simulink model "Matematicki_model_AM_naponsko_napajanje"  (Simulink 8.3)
settings: Solver=ode3  StartTime=0  StopTime=Tfinalno  FixedStep=Tsim  RelTol=1e-3
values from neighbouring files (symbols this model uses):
  A1 = [-Rsigma/Lsigma 0 Lm/(Tr*Lr*Lsigma) 0; 0 -Rsigma/Lsigma 0 Lm/(Tr*Lr*Lsigma); Lm/Tr 0 -1/Tr 0; 0 Lm/Tr 0 -1/Tr]    [Matematicki_model_AM_naponsko_napajanje_parametri.m]
  A2 = [0 1 0 0; -1 0 0 0; 0 0 0 1; 0 0 -1 0]    [Matematicki_model_AM_naponsko_napajanje_parametri.m]
  A3 = [0 0 0 Lm/(Lr*Lsigma); 0 0 -Lm/(Lr*Lsigma) 0; 0 0 0 -1; 0 0 1 0]    [Matematicki_model_AM_naponsko_napajanje_parametri.m]
  Am = [-Kfv*p/J -Kel*p/J; 1 0]    [Matematicki_model_AM_naponsko_napajanje_parametri.m]
  B = [1/Lsigma 0; 0 1/Lsigma; 0 0; 0 0]    [Matematicki_model_AM_naponsko_napajanje_parametri.m]
  Bm = [p/J -p/J; 0 0]    [Matematicki_model_AM_naponsko_napajanje_parametri.m]
  Kp = 0.1    [Matematicki_model_AM_naponsko_napajanje_parametri.m]
  Lm = 0.422    [Matematicki_model_AM_naponsko_napajanje_parametri.m]
  Lr = Lxr+Lm    (= 0.462)    [Matematicki_model_AM_naponsko_napajanje_parametri.m]
  Lsigma = Ls*sigm    (= 0.0765367965368)    [Matematicki_model_AM_naponsko_napajanje_parametri.m]
  Mopt = 2    [Matematicki_model_AM_naponsko_napajanje_parametri.m]
  p = 2    [Matematicki_model_AM_naponsko_napajanje_parametri.m]
  Tn = 10*Tr    (= 0.733333333333)    [Matematicki_model_AM_naponsko_napajanje_parametri.m]
  topt = 1    [Matematicki_model_AM_naponsko_napajanje_parametri.m]
  TROUGAO_ZVEZDA = 0    [Matematicki_model_AM_naponsko_napajanje_parametri.m]
  Tsim = Tpwm/16    (= 3.125e-06)    [Matematicki_model_AM_naponsko_napajanje_parametri.m]
  U_f = Vm/ws    [Matematicki_model_AM_naponsko_napajanje_parametri.m]
  Vm = sqrt(2)*Veff    [Matematicki_model_AM_naponsko_napajanje_parametri.m]
  wk = 2*pi()*50    [Matematicki_model_AM_naponsko_napajanje_parametri.m]
  wref = ws    [Matematicki_model_AM_naponsko_napajanje_parametri.m]
  ws = 2*pi()*fs    [Matematicki_model_AM_naponsko_napajanje_parametri.m]
libraries: simulink x1

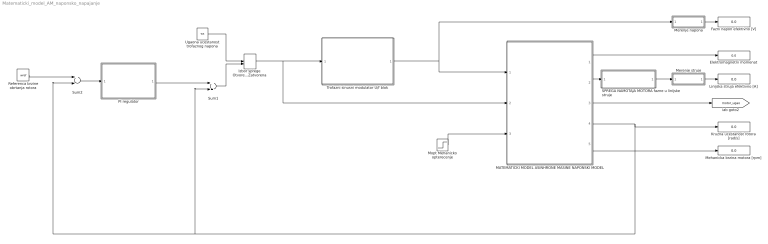
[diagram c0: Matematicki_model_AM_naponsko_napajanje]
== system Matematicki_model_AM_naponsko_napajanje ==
  Elektromagnetni momenat : Display
  Fazni napon efektivno [V] : Display
  Izbor sprege Otvorena / Zatvorena : ManualSwitch  CurrentSetting=0
  Kruzna ucestanost rotora [rad/s] : Display
  Linijska struja efektivno [A] : Display
  MATEMATICKI MODEL ASINHRONE MASINE NAPONSKI MODEL : Subsystem
  Mehanicka brzina motora [rpm] : Display
  Merenje napona : Subsystem
  Merenje struje : Subsystem
  Mopt Mehanicko opterecenje : Step  Time=4*topt  After=Mopt  SampleTime=Tsim
  PI regulator : Subsystem
  Referenca brzine obrtanja rotora : Constant  Value=wref  SampleTime=Tsim
  "SPREGA NAMOTAJA MOTORA fazne u linijske struje " : Subsystem
  Sum1 : Sum  SampleTime=Tsim
  Sum2 : Sum  Inputs=+-  SampleTime=Tsim
  Trofazni sinusni modulator U/f blok : Subsystem
  Ugaona ucestanost trofaznog napona : Constant  Value=ws  SampleTime=Tsim
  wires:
  Mopt Mehanicko opterecenje/1 -> MATEMATICKI MODEL ASINHRONE MASINE NAPONSKI MODEL/3(Mopt)
  MATEMATICKI MODEL ASINHRONE MASINE NAPONSKI MODEL/1(M_el) -> Elektromagnetni momenat/1
  MATEMATICKI MODEL ASINHRONE MASINE NAPONSKI MODEL/5(Brzina meh [o/min]) -> Mehanicka brzina motora [rpm]/1
  MATEMATICKI MODEL ASINHRONE MASINE NAPONSKI MODEL/3(ugao rot_el) -> [motor_ugao]
  Merenje napona/1(Us_eff) -> Fazni napon efektivno [V]/1
  Merenje struje/1(Is_eff) -> Linijska struja efektivno [A]/1
  "SPREGA NAMOTAJA MOTORA fazne u linijske struje "/1("Is_abc  invertor ") -> Merenje struje/1(Is_abc)
  MATEMATICKI MODEL ASINHRONE MASINE NAPONSKI MODEL/2(Is_abc) -> "SPREGA NAMOTAJA MOTORA fazne u linijske struje "/1(Is_abc fazno)
  MATEMATICKI MODEL ASINHRONE MASINE NAPONSKI MODEL/4(wr_el) -> Sum1/2, Sum2/2, Kruzna ucestanost rotora [rad/s]/1
  Ugaona ucestanost trofaznog napona/1 -> Izbor sprege Otvorena / Zatvorena/1
  Izbor sprege Otvorena / Zatvorena/1 -> MATEMATICKI MODEL ASINHRONE MASINE NAPONSKI MODEL/2(W_dq), Trofazni sinusni modulator U/f blok/1(ws)
  Sum1/1 -> Izbor sprege Otvorena / Zatvorena/2
  Referenca brzine obrtanja rotora/1 -> Sum2/1
  Sum2/1 -> PI regulator/1(e)
  PI regulator/1(wk) -> Sum1/1
  Trofazni sinusni modulator U/f blok/1(PWM) -> Merenje napona/1(Us_abc), MATEMATICKI MODEL ASINHRONE MASINE NAPONSKI MODEL/1(Us_abc)

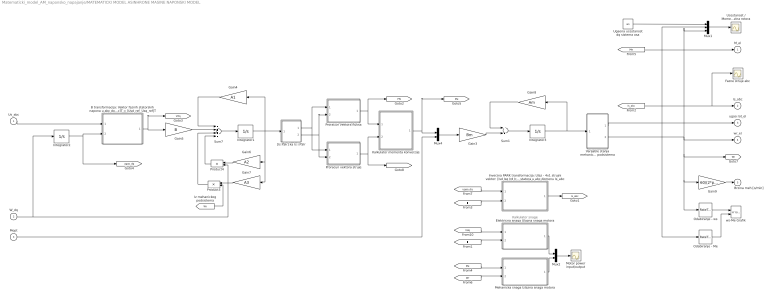
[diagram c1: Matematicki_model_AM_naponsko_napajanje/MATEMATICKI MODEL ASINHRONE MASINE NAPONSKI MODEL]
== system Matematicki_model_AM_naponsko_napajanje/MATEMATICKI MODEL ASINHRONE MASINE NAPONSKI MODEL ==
  note: Kalkulator snage
  Us_abc : Inport
  W_dq : Inport  Port=2
  Mopt : Inport  Port=3
  B transformacija: Vektor faznih statorskih napona u abc domenu u vektor napona u dq referentnom sistemu - [Usa  Usb Usc]T = [Usd_ref  Usq_ref]T : Subsystem
  Elektricna snaga Ulazna snaga motora : Subsystem
  Fazne struje abc : Scope
  Gain3 : Gain  Gain=Bm  Multiplication=Matrix(K*u) (u vector)  SampleTime=Tsim
  Gain4 : Gain  Gain=A1  Multiplication=Matrix(K*u) (u vector)  SampleTime=Tsim
  Gain5 : Gain  Gain=B  Multiplication=Matrix(K*u) (u vector)  SampleTime=Tsim
  Gain6 : Gain  Gain=A2  Multiplication=Matrix(K*u) (u vector)  SampleTime=Tsim
  Gain7 : Gain  Gain=A3  Multiplication=Matrix(K*u) (u vector)  SampleTime=Tsim
  Gain8 : Gain  Gain=Am  Multiplication=Matrix(K*u) (u vector)  SampleTime=Tsim
  Gain9 : Gain  Gain=60/(2*pi()*p)  SampleTime=Tsim
  Integrator1 : Integrator  InitialCondition=[0,0,0,0]
  Integrator2 : Integrator
  Integrator3 : Integrator  InitialCondition=[0,0]
  Inverzna PARK transformacija: Ulaz - 4x1 strujni vektor: [Isd Isq Ird Irq]T Izlaz - vektor struje statora u abc domenu Is_abc : Subsystem
  Kalkulator momenta konverzije : Subsystem
  Mehanicka snaga Izlazna snaga motora : Subsystem
  Motor power input/output : Scope
  Mux1 : Mux  Inputs=3
  Mux2 : Mux  Inputs=2
  Mux4 : Mux  Inputs=2
  Odabiranje - Me : RateTransition  OutPortSampleTime=100*Tsim
  Odabiranje - ws : RateTransition  OutPortSampleTime=100*Tsim
  Product3 : Product  SampleTime=Tsim
  Product4 : Product  SampleTime=Tsim
  Proracun vektora fluksa : Subsystem
  Proracun vektora struje : Subsystem
  Sum1 : Sum  SampleTime=Tsim
  Sum7 : Sum  Inputs=++++  SampleTime=Tsim
  Ucestanost / Momenat / Brzina rotora : Scope
  Ugaona ucestanost dq sistema osa : Constant  Value=ws  SampleTime=Tsim
  Varijable stanja mehanickog podsistema : Subsystem
  "[Is PSIr] ka Is i PSIr" : Subsystem
  ws-Me Grafik : simulink/Sinks/XY Graph  xmin=-400  xmax=400  ymin=-20  ymax=20  st=100*Tsim
  M_el : Outport  InitialOutput=0
  Is_abc : Outport  Port=2  InitialOutput=0
  ugao rot_el : Outport  Port=3  InitialOutput=0
  wr_el : Outport  Port=4  InitialOutput=0
  Brzina meh [o/min] : Outport  Port=5  InitialOutput=0
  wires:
  Us_abc/1 -> B transformacija: Vektor faznih statorskih napona u abc domenu u vektor napona u dq referentnom sistemu - [Usa  Usb Usc]T = [Usd_ref  Usq_ref]T/1(Us_abc)
  Integrator1/1 -> Gain4/1, Gain7/1, Gain6/1, "[Is PSIr] ka Is i PSIr"/1(X1)
  [Wr] -> Product3/2
  Product3/1 -> Sum7/3
  Gain7/1 -> Product3/1
  Gain6/1 -> Product4/1
  Sum7/1 -> Integrator1/1
  Gain4/1 -> Sum7/1
  Gain5/1 -> Sum7/2
  W_dq/1 -> Integrator2/1, Product4/2
  Integrator2/1 -> [ugao_dq], B transformacija: Vektor faznih statorskih napona u abc domenu u vektor napona u dq referentnom sistemu - [Usa  Usb Usc]T = [Usd_ref  Usq_ref]T/2(ugao_dq)
  [I] -> Inverzna PARK transformacija: Ulaz - 4x1 strujni vektor: [Isd Isq Ird Irq]T Izlaz - vektor struje statora u abc domenu Is_abc/2(I)
  B transformacija: Vektor faznih statorskih napona u abc domenu u vektor napona u dq referentnom sistemu - [Usa  Usb Usc]T = [Usd_ref  Usq_ref]T/1(Us_dq) -> Gain5/1, [Vdq]
  [I] -> Elektricna snaga Ulazna snaga motora/2(Is_dq)
  Elektricna snaga Ulazna snaga motora/1(Pel) -> Mux2/1
  [Me] -> Mehanicka snaga Izlazna snaga motora/1(Me)
  [Wr] -> Mehanicka snaga Izlazna snaga motora/2(Wr)
  Mux2/1 -> Motor power input/output/1
  Mehanicka snaga Izlazna snaga motora/1(Pmeh) -> Mux2/2
  [Vdq] -> Elektricna snaga Ulazna snaga motora/1(Vs_dq)
  Product4/1 -> Sum7/4
  "[Is PSIr] ka Is i PSIr"/1(Is) -> Proracun vektora struje/1(Is), Proracun vektora fluksa/1(Is)
  "[Is PSIr] ka Is i PSIr"/2(PSIr) -> Proracun vektora struje/2(PSIr), Proracun vektora fluksa/2(PSIr)
  Proracun vektora fluksa/1(PSI) -> [PSI], Kalkulator momenta konverzije/1(PSI)
  Proracun vektora struje/1(I) -> [I], Kalkulator momenta konverzije/2(I)
  Kalkulator momenta konverzije/1(Me) -> [Me], Mux4/1
  Mopt/1 -> Mux4/2
  [Me] -> M_el/1, Mux1/2, Odabiranje - Me/1
  Varijable stanja mehanickog podsistema/1(theta) -> ugao rot_el/1
  Varijable stanja mehanickog podsistema/2(w) -> Odabiranje - ws/1, Gain9/1, [Wr], wr_el/1, Mux1/3
  Gain9/1 -> Brzina meh [o/min]/1
  Inverzna PARK transformacija: Ulaz - 4x1 strujni vektor: [Isd Isq Ird Irq]T Izlaz - vektor struje statora u abc domenu Is_abc/1(Is_abc) -> [Is_abc]
  Mux4/1 -> Gain3/1
  Gain3/1 -> Sum1/2
  Sum1/1 -> Integrator3/1
  Gain8/1 -> Sum1/1
  Integrator3/1 -> Varijable stanja mehanickog podsistema/1(X2), Gain8/1
  [Is_abc] -> Is_abc/1, Fazne struje abc/1
  [ugao_dq] -> Inverzna PARK transformacija: Ulaz - 4x1 strujni vektor: [Isd Isq Ird Irq]T Izlaz - vektor struje statora u abc domenu Is_abc/1(ugao_dq)
  Mux1/1 -> Ucestanost / Momenat / Brzina rotora/1
  Odabiranje - ws/1 -> ws-Me Grafik/1
  Odabiranje - Me/1 -> ws-Me Grafik/2
  Ugaona ucestanost dq sistema osa/1 -> Mux1/1

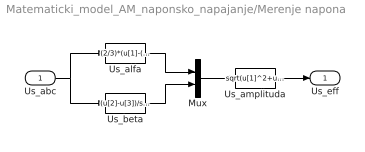
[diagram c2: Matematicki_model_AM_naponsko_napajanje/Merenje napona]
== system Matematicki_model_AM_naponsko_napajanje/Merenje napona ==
  Us_abc : Inport
  Mux : Mux  Inputs=2
  Us_alfa : Fcn  Expr=(2/3)*(u[1]-(u[2]+u[3])/2)  SampleTime=Tsim
  Us_amplituda : Fcn  Expr=sqrt(u[1]^2+u[2]^2)  SampleTime=Tsim
  Us_beta : Fcn  Expr=(u[2]-u[3])/sqrt(3)  SampleTime=Tsim
  Us_eff : Outport
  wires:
  Us_abc/1 -> Us_beta/1, Us_alfa/1
  Us_alfa/1 -> Mux/1
  Us_beta/1 -> Mux/2
  Mux/1 -> Us_amplituda/1
  Us_amplituda/1 -> Us_eff/1

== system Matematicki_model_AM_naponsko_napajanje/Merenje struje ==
  Is_abc : Inport
  Is_alfa : Fcn  Expr=(2/3)*(u[1]-(u[2]+u[3])/2)  SampleTime=Tsim
  Is_amplituda : Fcn  Expr=sqrt(u[1]^2+u[2]^2)/sqrt(2)  SampleTime=Tsim
  Is_beta : Fcn  Expr=(u[2]-u[3])/sqrt(3)  SampleTime=Tsim
  Mux : Mux  Inputs=2
  Is_eff : Outport
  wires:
  Is_amplituda/1 -> Is_eff/1
  Mux/1 -> Is_amplituda/1
  Is_beta/1 -> Mux/2
  Is_alfa/1 -> Mux/1
  Is_abc/1 -> Is_alfa/1, Is_beta/1

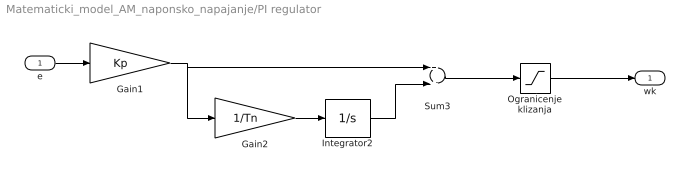
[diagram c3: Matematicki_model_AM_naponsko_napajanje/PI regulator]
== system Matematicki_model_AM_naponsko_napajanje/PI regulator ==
  e : Inport
  Gain1 : Gain  Gain=Kp  SampleTime=Tsim
  Gain2 : Gain  Gain=1/Tn  SampleTime=Tsim
  Integrator2 : Integrator  InitialCondition=[0]
  Ogranicenje klizanja : Saturate  UpperLimit=wk  LowerLimit=-wk  SampleTime=Tsim
  Sum3 : Sum  SampleTime=Tsim
  wk : Outport
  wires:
  Gain1/1 -> Sum3/1, Gain2/1
  e/1 -> Gain1/1
  Sum3/1 -> Ogranicenje klizanja/1
  Integrator2/1 -> Sum3/2
  Gain2/1 -> Integrator2/1
  Ogranicenje klizanja/1 -> wk/1

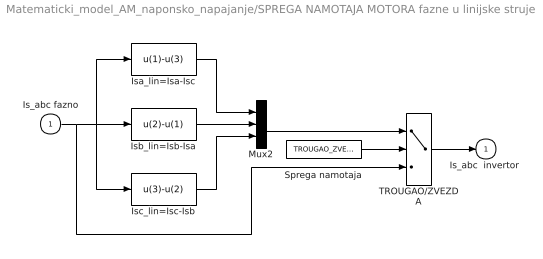
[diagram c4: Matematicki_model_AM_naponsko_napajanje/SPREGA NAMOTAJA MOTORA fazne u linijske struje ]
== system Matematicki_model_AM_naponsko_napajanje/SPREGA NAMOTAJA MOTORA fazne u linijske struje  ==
  Is_abc fazno : Inport
  Isa_lin=Isa-Isc : Fcn  Expr=u(1)-u(3)  SampleTime=Tsim
  Isb_lin=Isb-Isa : Fcn  Expr=u(2)-u(1)  SampleTime=Tsim
  Isc_lin=Isc-Isb : Fcn  Expr=u(3)-u(2)  SampleTime=Tsim
  Mux2 : Mux  Inputs=3
  Sprega namotaja : Constant  Value=TROUGAO_ZVEZDA
  TROUGAO/ZVEZDA : Switch  Threshold=0.1  SampleTime=Tsim
  "Is_abc  invertor " : Outport  InitialOutput=0
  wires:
  Isc_lin=Isc-Isb/1 -> Mux2/3
  Isb_lin=Isb-Isa/1 -> Mux2/2
  Isa_lin=Isa-Isc/1 -> Mux2/1
  Is_abc fazno/1 -> Isc_lin=Isc-Isb/1, Isb_lin=Isb-Isa/1, Isa_lin=Isa-Isc/1, TROUGAO/ZVEZDA/3
  TROUGAO/ZVEZDA/1 -> "Is_abc  invertor "/1
  Mux2/1 -> TROUGAO/ZVEZDA/1
  Sprega namotaja/1 -> TROUGAO/ZVEZDA/2

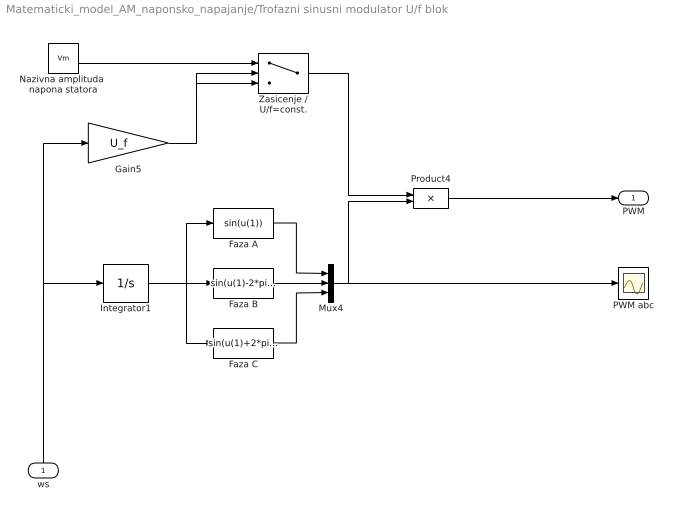
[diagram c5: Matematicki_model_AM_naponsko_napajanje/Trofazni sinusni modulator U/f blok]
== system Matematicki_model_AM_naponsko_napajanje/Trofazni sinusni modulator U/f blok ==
  ws : Inport
  Faza A : Fcn  Expr=sin(u(1))  SampleTime=Tsim
  Faza B : Fcn  Expr=sin(u(1)-2*pi()/3)  SampleTime=Tsim
  Faza C : Fcn  Expr=sin(u(1)+2*pi()/3)  SampleTime=Tsim
  Gain5 : Gain  Gain=U_f  SampleTime=Tsim
  Integrator1 : Integrator  InitialCondition=[0]
  Mux4 : Mux  Inputs=3
  Nazivna amplituda  napona statora : Constant  Value=Vm  SampleTime=Tsim
  PWM abc : Scope
  Product4 : Product  SampleTime=Tsim
  Zasicenje / U/f=const. : Switch  Criteria=u2 > Threshold  Threshold=Vm  SampleTime=Tsim
  PWM : Outport
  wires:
  Faza B/1 -> Mux4/2
  Faza A/1 -> Mux4/1
  Faza C/1 -> Mux4/3
  Gain5/1 -> Zasicenje / U/f=const./3, Zasicenje / U/f=const./2
  Nazivna amplituda  napona statora/1 -> Zasicenje / U/f=const./1
  Mux4/1 -> Product4/2, PWM abc/1
  Zasicenje / U/f=const./1 -> Product4/1
  Product4/1 -> PWM/1
  ws/1 -> Integrator1/1, Gain5/1
  Integrator1/1 -> Faza C/1, Faza B/1, Faza A/1

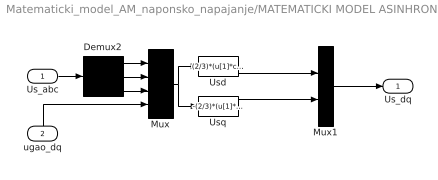
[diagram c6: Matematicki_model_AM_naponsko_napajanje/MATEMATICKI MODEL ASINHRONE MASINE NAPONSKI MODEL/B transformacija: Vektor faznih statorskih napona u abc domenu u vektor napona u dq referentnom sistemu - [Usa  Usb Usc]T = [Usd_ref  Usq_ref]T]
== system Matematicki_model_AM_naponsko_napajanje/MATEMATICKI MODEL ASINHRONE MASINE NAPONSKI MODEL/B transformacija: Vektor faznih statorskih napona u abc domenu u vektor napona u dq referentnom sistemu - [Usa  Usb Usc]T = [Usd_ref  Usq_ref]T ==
  Us_abc : Inport
  ugao_dq : Inport  Port=2
  Demux2 : Demux  Outputs=3
  Mux : Mux
  Mux1 : Mux  Inputs=2
  Usd : Fcn  Expr=(2/3)*(u[1]*cos(u[4])+u[2]*cos(u[4]-2*pi/3)+u[3]*cos(u[4]-4*pi/3))  SampleTime=Tsim
  Usq : Fcn  Expr=-(2/3)*(u[1]*sin(u[4])+u[2]*sin(u[4]-2*pi/3)+u[3]*sin(u[4]-4*pi/3))  SampleTime=Tsim
  Us_dq : Outport
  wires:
  Usd/1 -> Mux1/1
  Usq/1 -> Mux1/2
  Mux/1 -> Usq/1, Usd/1
  Demux2/2 -> Mux/2
  Demux2/3 -> Mux/3
  Demux2/1 -> Mux/1
  ugao_dq/1 -> Mux/4
  Us_abc/1 -> Demux2/1
  Mux1/1 -> Us_dq/1

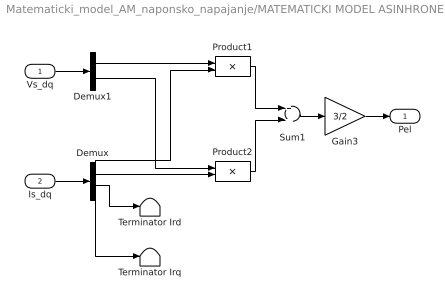
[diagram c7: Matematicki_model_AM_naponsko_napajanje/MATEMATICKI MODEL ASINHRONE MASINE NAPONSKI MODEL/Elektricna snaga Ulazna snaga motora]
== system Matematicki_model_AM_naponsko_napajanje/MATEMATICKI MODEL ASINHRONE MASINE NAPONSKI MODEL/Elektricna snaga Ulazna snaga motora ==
  Vs_dq : Inport
  Is_dq : Inport  Port=2
  Demux : Demux
  Demux1 : Demux  Outputs=2
  Gain3 : Gain  Gain=3/2  SampleTime=Tsim
  Product1 : Product  SampleTime=Tsim
  Product2 : Product  SampleTime=Tsim
  Sum1 : Sum  SampleTime=Tsim
  Terminator Ird : Terminator
  Terminator Irq : Terminator
  Pel : Outport
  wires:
  Sum1/1 -> Gain3/1
  Product2/1 -> Sum1/2
  Product1/1 -> Sum1/1
  Demux/2 -> Product2/2
  Demux1/2 -> Product2/1
  Demux/1 -> Product1/2
  Demux1/1 -> Product1/1
  Demux/3 -> Terminator Ird/1
  Demux/4 -> Terminator Irq/1
  Vs_dq/1 -> Demux1/1
  Gain3/1 -> Pel/1
  Is_dq/1 -> Demux/1

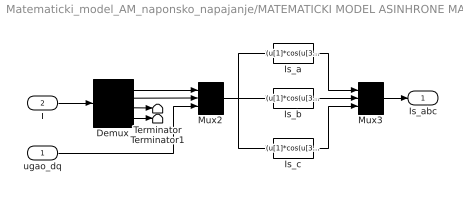
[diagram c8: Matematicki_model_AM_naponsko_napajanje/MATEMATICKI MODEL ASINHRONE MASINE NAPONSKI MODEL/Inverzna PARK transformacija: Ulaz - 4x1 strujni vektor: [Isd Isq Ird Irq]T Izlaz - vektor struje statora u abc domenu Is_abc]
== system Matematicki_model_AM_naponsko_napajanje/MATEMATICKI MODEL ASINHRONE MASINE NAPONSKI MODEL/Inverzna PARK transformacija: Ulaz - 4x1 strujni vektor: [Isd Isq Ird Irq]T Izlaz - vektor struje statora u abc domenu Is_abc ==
  ugao_dq : Inport
  I : Inport  Port=2
  Demux : Demux
  Is_a : Fcn  Expr=(u[1]*cos(u[3])-u[2]*sin(u[3]))  SampleTime=Tsim
  Is_b : Fcn  Expr=(u[1]*cos(u[3]-2*pi/3)-u[2]*sin(u[3]-2*pi/3))  SampleTime=Tsim
  Is_c : Fcn  Expr=(u[1]*cos(u[3]-4*pi/3)-u[2]*sin(u[3]-4*pi/3))  SampleTime=Tsim
  Mux2 : Mux  Inputs=3
  Mux3 : Mux  Inputs=3
  Terminator : Terminator
  Terminator1 : Terminator
  Is_abc : Outport
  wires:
  ugao_dq/1 -> Mux2/3
  Mux3/1 -> Is_abc/1
  I/1 -> Demux/1
  Mux2/1 -> Is_c/1, Is_a/1, Is_b/1
  Is_a/1 -> Mux3/1
  Is_b/1 -> Mux3/2
  Is_c/1 -> Mux3/3
  Demux/3 -> Terminator/1
  Demux/4 -> Terminator1/1
  Demux/1 -> Mux2/1
  Demux/2 -> Mux2/2

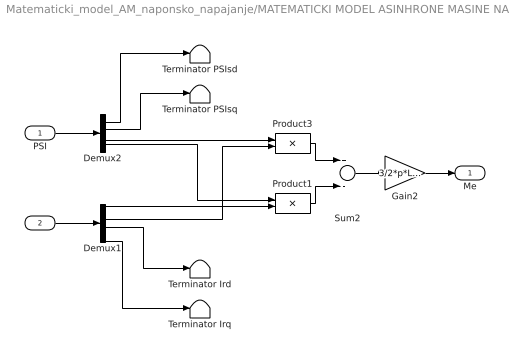
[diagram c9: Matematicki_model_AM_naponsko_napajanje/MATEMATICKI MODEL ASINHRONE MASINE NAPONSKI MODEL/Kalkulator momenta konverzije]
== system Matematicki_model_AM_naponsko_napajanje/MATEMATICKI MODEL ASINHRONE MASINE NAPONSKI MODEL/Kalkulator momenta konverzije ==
  PSI : Inport
  I : Inport  Port=2
  Demux1 : Demux
  Demux2 : Demux
  Gain2 : Gain  Gain=3/2*p*Lm/Lr  SampleTime=Tsim
  Product1 : Product  SampleTime=Tsim
  Product3 : Product  SampleTime=Tsim
  Sum2 : Sum  Inputs=+-  SampleTime=Tsim
  Terminator Ird : Terminator
  Terminator Irq : Terminator
  Terminator PSIsd : Terminator
  Terminator PSIsq : Terminator
  Me : Outport
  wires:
  PSI/1 -> Demux2/1
  Demux2/1 -> Terminator PSIsd/1
  Demux2/2 -> Terminator PSIsq/1
  Demux1/1 -> Product1/2
  Demux1/2 -> Product3/2
  I/1 -> Demux1/1
  Demux2/4 -> Product1/1
  Demux2/3 -> Product3/1
  Product3/1 -> Sum2/1
  Product1/1 -> Sum2/2
  Gain2/1 -> Me/1
  Sum2/1 -> Gain2/1
  Demux1/3 -> Terminator Ird/1
  Demux1/4 -> Terminator Irq/1

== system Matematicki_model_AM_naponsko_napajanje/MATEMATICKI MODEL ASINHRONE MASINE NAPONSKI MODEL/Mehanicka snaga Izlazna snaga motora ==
  note: Pmeh=Mel*Wr_el/P
  Me : Inport
  Wr : Inport  Port=2
  Gain11 : Gain  Gain=1/p  SampleTime=Tsim
  Product6 : Product  SampleTime=Tsim
  Pmeh : Outport
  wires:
  Product6/1 -> Gain11/1
  Me/1 -> Product6/1
  Gain11/1 -> Pmeh/1
  Wr/1 -> Product6/2

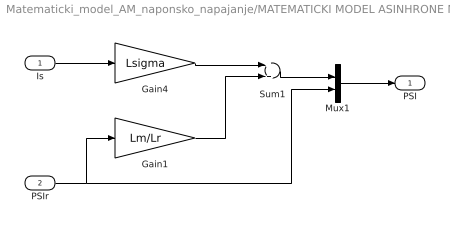
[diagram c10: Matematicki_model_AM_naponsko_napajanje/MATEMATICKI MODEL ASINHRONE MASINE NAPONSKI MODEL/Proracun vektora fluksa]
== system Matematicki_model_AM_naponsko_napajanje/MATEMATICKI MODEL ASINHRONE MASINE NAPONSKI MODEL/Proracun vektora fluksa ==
  Is : Inport
  PSIr : Inport  Port=2
  Gain1 : Gain  Gain=Lm/Lr  SampleTime=Tsim
  Gain4 : Gain  Gain=Lsigma  SampleTime=Tsim
  Mux1 : Mux  Inputs=2
  Sum1 : Sum  SampleTime=Tsim
  PSI : Outport
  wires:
  Is/1 -> Gain4/1
  Mux1/1 -> PSI/1
  PSIr/1 -> Gain1/1, Mux1/2
  Gain1/1 -> Sum1/2
  Gain4/1 -> Sum1/1
  Sum1/1 -> Mux1/1

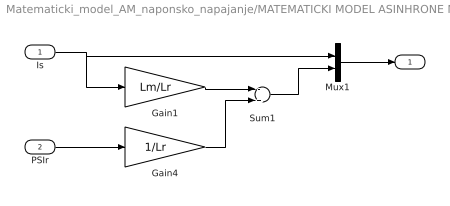
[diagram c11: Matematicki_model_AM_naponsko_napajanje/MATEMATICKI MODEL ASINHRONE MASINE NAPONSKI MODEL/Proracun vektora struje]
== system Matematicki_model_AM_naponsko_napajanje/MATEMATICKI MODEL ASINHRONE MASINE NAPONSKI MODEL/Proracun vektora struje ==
  Is : Inport
  PSIr : Inport  Port=2
  Gain1 : Gain  Gain=Lm/Lr  SampleTime=Tsim
  Gain4 : Gain  Gain=1/Lr  SampleTime=Tsim
  Mux1 : Mux  Inputs=2
  Sum1 : Sum  Inputs=-+  SampleTime=Tsim
  I : Outport
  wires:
  Is/1 -> Gain1/1, Mux1/1
  Mux1/1 -> I/1
  PSIr/1 -> Gain4/1
  Gain1/1 -> Sum1/1
  Gain4/1 -> Sum1/2
  Sum1/1 -> Mux1/2

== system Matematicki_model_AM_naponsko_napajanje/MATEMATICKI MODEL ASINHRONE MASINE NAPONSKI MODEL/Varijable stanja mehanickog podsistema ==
  X2 : Inport
  Demux2 : Demux  Outputs=2
  theta : Outport
  w : Outport  Port=2
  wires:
  X2/1 -> Demux2/1
  Demux2/2 -> theta/1
  Demux2/1 -> w/1

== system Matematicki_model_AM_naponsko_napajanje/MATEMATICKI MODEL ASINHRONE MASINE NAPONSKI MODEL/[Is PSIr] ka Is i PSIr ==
  X1 : Inport
  Demux2 : Demux
  Mux1 : Mux  Inputs=2
  Mux2 : Mux  Inputs=2
  Is : Outport
  PSIr : Outport  Port=2
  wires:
  Demux2/1 -> Mux1/1
  Demux2/4 -> Mux2/2
  X1/1 -> Demux2/1
  Mux1/1 -> Is/1
  Mux2/1 -> PSIr/1
  Demux2/3 -> Mux2/1
  Demux2/2 -> Mux1/2
